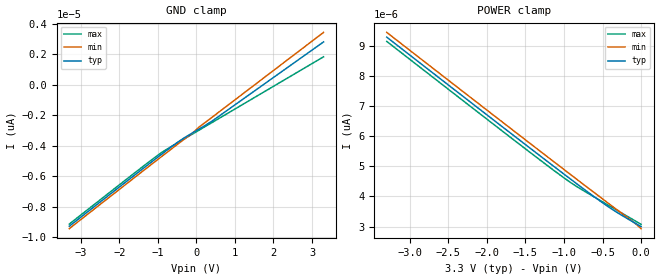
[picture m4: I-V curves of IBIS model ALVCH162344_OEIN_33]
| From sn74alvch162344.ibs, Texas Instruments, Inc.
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[Model]   ALVCH162344_OEIN_33
Model_type  Input
Vinl = 0.8
Vinh = 2.0
| variable   typ   min   max
C_comp   1.31pF   1.13pF   1.45pF
[Temperature Range]   40   100   -40
| Ambient temperature   25   85   -40
[Voltage range]   3.3   3   3.6
[GND Clamp]
| ALVCH162344_OEIN_33
|   Voltage   I(typ)   I(min)   I(max)
-3.3V     -9.28pA    -9.437pA   -9.14pA
-1.46V    -5.64pA    -5.797pA   -5.5pA
-865mV    -4.48pA    -4.63pA    -4.379pA
-370mV    -3.567pA   -3.671pA   -3.629pA
450mV     -2.299pA   -2.043pA   -2.406pA
3.3V      2.819pA    3.444pA    1.842pA
[POWER Clamp]
| ALVCH162344_OEIN_33
|   Voltage   I(typ)   I(min)   I(max)
-3.3V     9.28pA     9.437pA    9.14pA
-1.675V   6.063pA    6.221pA    5.921pA
-995mV    4.731pA    4.884pA    4.608pA
-810mV    4.374pA    4.522pA    4.29pA
-435mV    3.677pA    3.795pA    3.726pA
-105mV    3.158pA    3.165pA    3.234pA
0V        3.001pA    2.933pA    3.077pA
